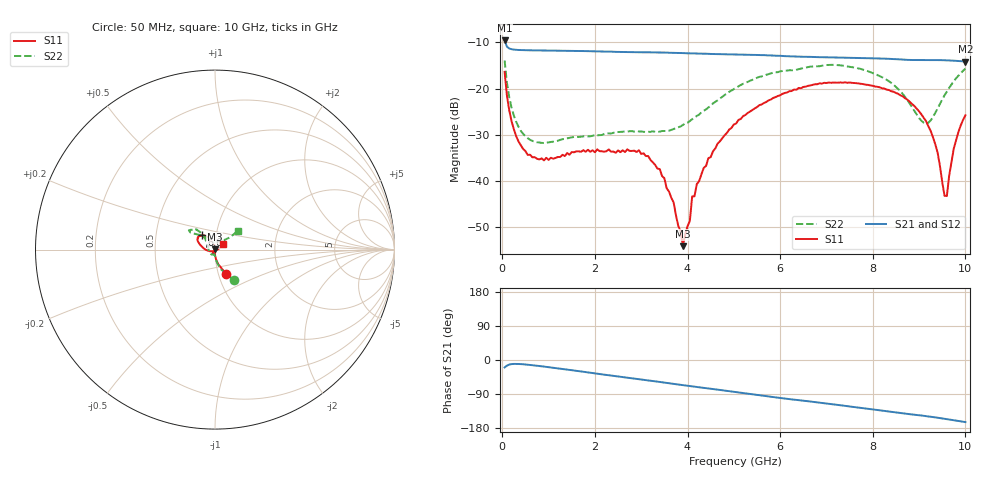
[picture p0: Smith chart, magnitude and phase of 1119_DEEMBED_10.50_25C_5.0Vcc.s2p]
!Hittite Microwave Corp.
!Digital Attenuator/PhaseShifter Rev 1.4.0
!Filename: C:\DATA\DATA\1119_DEEMBED_10.50_25C_5.0Vcc.s2p
!VNA ID: Agilent Technologies,N5224A,MY51441122,A.10.45.03
!Device type:
!2 Port Calibration.
!Temp(C): 25
!Lot Number:
!Serial Number:
!Operator:
!Misc:
!Attenuator:  10.500
# GHZ S DB R 50.0
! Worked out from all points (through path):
!   200 points, 50 MHz to 10 GHz, reference 50 ohm
!   highest |S21| = -9.57 dB at 50 MHz (marker M1); lowest = -14.1 dB at 10 GHz (marker M2)
!   group delay of S21, straight-line fit = 43.8 ps
!   lowest |S11| = -54.1 dB at 3.9 GHz (marker M3), VSWR 1.00, Z = 49.8 + j0.0693 ohm
!   |S11| at or under -10 dB: start of sweep to end of sweep
!   |S22| runs from -31.7 to -13.9 dB; largest |S21 - S12| = 0.00087
!   S11 on the Smith chart (normalised r, x): 50 MHz: 1.09, -0.31; 6.6 GHz: 0.86, +0.14; 10 GHz: 1.09, +0.06
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0.05  -16.37 -65.2  -9.57 -19.7  -9.57 -19.7  -13.90 -57.7
0.1  -21.50 -77.3  -10.91 -14.8  -10.91 -14.8  -18.67 -72.7
0.2  -27.05 -85.9  -11.46 -10.8  -11.47 -10.9  -24.10 -83.3
0.55  -34.34 -96.9  -11.69 -12.4  -11.69 -12.4  -30.71 -93.8
1.75  -33.30 -114.2  -11.86 -31.1  -11.86 -31.1  -30.31 -110.8
2.95  -33.30 -105.9  -12.12 -50.4  -12.12 -50.5  -29.24 -148.2
3.4  -37.38 -111.6  -12.17 -57.9  -12.18 -58.0  -29.27 -169.2
3.7  -44.63 -117.0  -12.23 -63.0  -12.24 -63.0  -28.75 174.8
3.9  -54.06 159.4  -12.30 -66.4  -12.30 -66.4  -27.84 163.8
4.05  -48.60 117.2  -12.35 -68.7  -12.36 -68.8  -27.00 155.3
4.1  -43.30 110.3  -12.36 -69.6  -12.37 -69.7  -26.60 153.1
4.35  -37.14 95.6  -12.44 -73.5  -12.45 -73.5  -24.78 142.1
5.05  -27.52 109.0  -12.59 -84.6  -12.61 -84.6  -19.78 129.5
6.6  -19.38 132.2  -13.12 -108.8  -13.14 -108.8  -15.34 139.8
6.7  -19.18 133.7  -13.14 -110.3  -13.15 -110.3  -15.20 140.2
8.35  -20.29 158.1  -13.55 -136.2  -13.55 -136.2  -18.40 136.7
9.15  -27.00 -173.9  -13.80 -148.1  -13.81 -148.1  -27.54 87.4
9.400001  -33.81 -151.8  -13.81 -152.3  -13.82 -152.3  -24.29 52.5
9.55  -43.17 -90.2  -13.85 -155.1  -13.86 -155.2  -21.42 43.2
9.6  -43.20 -41.1  -13.87 -156.1  -13.89 -156.1  -20.60 41.6
9.75  -32.91 15.0  -13.95 -159.0  -13.96 -159.0  -18.37 39.2
10  -25.76 35.2  -14.13 -163.8  -14.13 -163.8  -15.67 39.8
